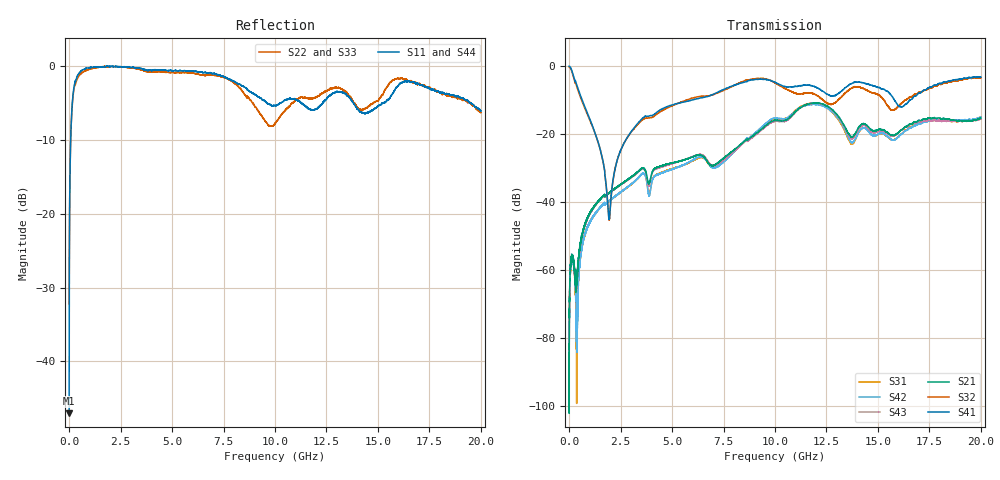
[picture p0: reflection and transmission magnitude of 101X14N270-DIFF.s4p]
!{101X14N270}
!Johanson Technology Inc.
!www.johansontechnology.com
!Test Board Conditions:
!Substrate Type  RO4350B
!Substrate Thickness  10 mil
!Substrate Dk  3.66
!TL Type: GCPW
!TL Trace Width  20 mil
!TL Gap  15 mil
!PART MODE DIFFERENTIAL
!DUT TOPOLOGY	DIFFERENTIAL 4-PORT
!Mounting Pad LxW  20x35 mil
# MHz S  dB  R 50
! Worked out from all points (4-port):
!   20001 points, 300 kHz to 20 GHz, reference 50 ohm
!   strongest paths, dB at 300 kHz, 5 GHz, 10 GHz, 15 GHz, 20 GHz:
!     S41: 0.0, -11.4, -4.7, -6.3, -3.2
!     S32: -0.3, -11.7, -4.9, -8.4, -3.4
!     S21: -84.2, -28.5, -15.9, -18.7, -15.3
!     S43: -81.0, -28.7, -16.2, -19.2, -15.5
!     S42: -75.2, -30.3, -15.2, -20.1, -15.0
!     S31: -98.9, -30.2, -15.5, -20.2, -15.0
!   lowest |S11| = -47.0 dB at 300 kHz (marker M1), VSWR 1.01, Z = 50.1 - j0.432 ohm
!   |S11| at or under -10 dB: start of sweep to 76.1 MHz
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0.3  -47.02 -75.4  -75.44 52.8  -83.78 157.1  -0.04 0.2
     -84.16 -62.3  -32.22 -9.3  -0.25 0.1  -79.45 -81.6
     -98.86 170.1  -0.27 0.2  -31.85 -11.0  -80.08 135.2
     -0.03 0.3  -75.22 72.2  -81.05 120.9  -47.70 -81.3
257.296  -2.53 -141.5  -59.73 15.6  -61.24 -7.3  -3.76 -50.9
         -59.52 16.3  -2.75 -141.4  -4.18 -51.4  -59.76 -12.8
         -60.82 -14.4  -4.19 -51.5  -2.95 -141.4  -60.04 13.7
         -3.77 -50.9  -60.18 -12.9  -59.75 9.0  -2.48 -141.6
1946.271  -0.06 168.9  -37.21 77.0  -39.60 76.8  -45.09 -8.0
          -37.20 77.0  -0.08 170.3  -45.10 -9.4  -39.62 77.5
          -39.66 76.8  -45.13 -9.5  -0.06 170.8  -37.39 77.8
          -44.98 -8.2  -39.71 76.9  -37.35 77.9  -0.08 170.2
3019.255  -0.20 162.2  -32.54 63.7  -34.74 60.2  -19.17 68.6
          -32.58 63.7  -0.24 163.2  -19.37 67.8  -34.60 61.6
          -34.73 60.6  -19.36 67.9  -0.29 164.2  -32.65 65.1
          -19.23 68.7  -34.62 61.0  -32.71 64.9  -0.08 164.0
5713.214  -0.66 128.6  -27.28 22.0  -28.69 14.3  -10.30 40.4
          -27.32 21.9  -0.88 136.4  -9.96 45.5  -28.49 17.7
          -28.70 14.2  -9.94 45.5  -0.96 137.8  -27.17 27.7
          -10.36 40.6  -28.54 17.8  -27.26 27.9  -0.57 137.6
11661.12  -5.82 111.3  -11.07 113.4  -11.00 118.1  -5.60 -33.0
          -11.08 113.4  -4.39 119.5  -7.83 -39.9  -11.30 116.6
          -11.00 118.0  -7.84 -39.9  -4.54 124.1  -11.06 115.7
          -5.62 -33.0  -11.32 116.6  -11.08 115.8  -5.54 112.7
20000  -6.08 39.8  -15.32 -117.0  -15.01 -119.1  -3.18 -65.6
       -15.31 -117.2  -6.30 47.0  -3.46 -62.9  -14.98 -119.8
       -14.97 -118.4  -3.43 -62.1  -6.47 55.5  -15.49 -109.2
       -3.17 -65.3  -15.00 -119.3  -15.54 -109.4  -5.86 46.6
